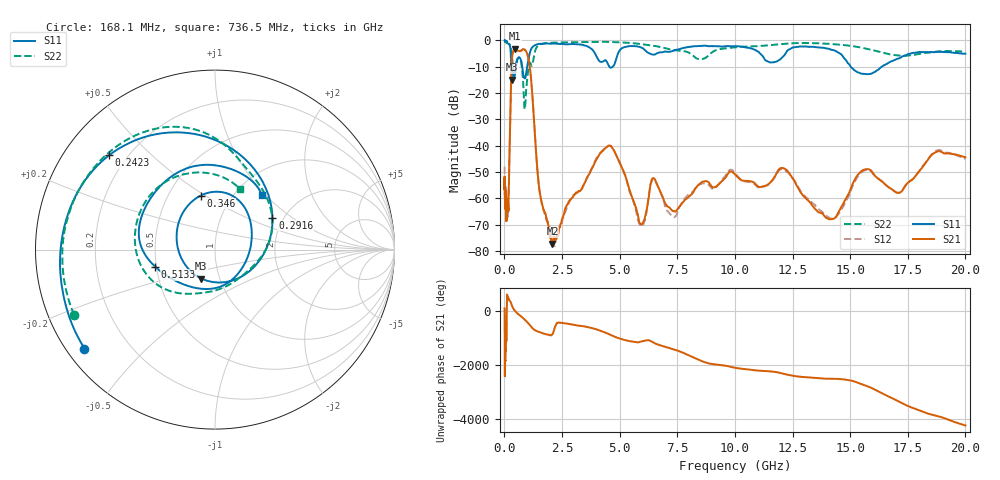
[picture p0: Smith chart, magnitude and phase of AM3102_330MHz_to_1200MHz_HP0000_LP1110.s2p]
! Date/Time: Tue, Sep 11, 2018 5:09 PM
! Network Analyzer: Agilent Technologies E8362B Rev: A.07.50.63
! Sweep from 0.010 to 20.000 GHz, 1601 Points, Sweep Type: LOG
! Power Supply: 4.950 V, 0.001 A
# Hz S DB R 50
!freq MagS11 AngS11 MagS21 AngS21 MagS12 AngS12 MagS22 AngS22
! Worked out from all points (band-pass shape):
!   1601 points, 10 MHz to 20 GHz, reference 50 ohm
!   highest |S21| = -3.10 dB at 464.5 MHz (marker M1); lowest = -77.2 dB at 2.084 GHz (marker M2)
!   |S21| within 3 dB of the highest: 337.5 MHz to 1.025 GHz (687.7 MHz wide, 101 % of centre)
!   lowest |S11| = -15.0 dB at 314.7 MHz (marker M3), VSWR 1.43, Z = 40.9 - j13.6 ohm
!   |S11| at or under -10 dB: 362.8 MHz to 503.8 MHz (141 MHz wide, 32.6 % of centre); 772.7 MHz to 987.7 MHz (215 MHz wide, 24.4 % of centre); 15.03 GHz to 16.37 GHz (1.346 GHz wide, 8.57 % of centre)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
!   |S22| runs from -26.1 to -0.3 dB; largest |S21 - S12| = 0.012
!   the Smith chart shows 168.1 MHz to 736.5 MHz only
!   S11 on the Smith chart (normalised r, x): 168.1 MHz: 0.05, -0.34; 242.3 MHz: 0.13, +0.38; 291.6 MHz: 1.75, +0.72; 346 MHz: 0.72, +0.48; 513.3 MHz: 0.49, -0.11; 736.5 MHz: 1.32, +0.95
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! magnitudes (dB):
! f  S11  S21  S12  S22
! 10 MHz  0.0  -56.5  -48.0  -0.3
! 35.55 MHz  0.0  -61.9  -59.3  -0.6
! 126.4 MHz  -0.4  -62.5  -65.8  -1.1
! 168.1 MHz  -0.8  -63.9  -64.7  -1.3
! 242.3 MHz  -2.0  -34.4  -34.4  -1.8
! 291.6 MHz  -8.7  -13.9  -14.0  -3.4
! 314.7 MHz  -15.0  -8.3  -8.3  -5.4
! 346 MHz  -10.1  -5.6  -5.7  -7.5
! 447.2 MHz  -13.6  -3.1  -3.2  -13.2
! 464.5 MHz  -12.8  -3.1  -3.1  -12.5
! 513.3 MHz  -9.2  -3.3  -3.4  -9.4
! 736.5 MHz  -8.0  -3.8  -3.9  -8.8
! 882.2 MHz  -14.5  -3.5  -3.6  -26.1
! 1.098 GHz  -5.0  -9.7  -9.6  -8.5
! 1.59 GHz  -1.4  -60.4  -60.6  -1.4
! 2.084 GHz  -1.2  -77.2  -78.1  -0.8
! 4.457 GHz  -8.3  -40.4  -40.3  -0.5
! 5.652 GHz  -2.1  -62.3  -62.8  -1.1
! 12.09 GHz  -6.1  -48.5  -49.0  -1.3
! 14.07 GHz  -3.2  -67.9  -67.3  -1.3
! 15.55 GHz  -12.7  -49.3  -49.8  -2.8
! 20 GHz  -5.0  -44.4  -45.1  -4.2
